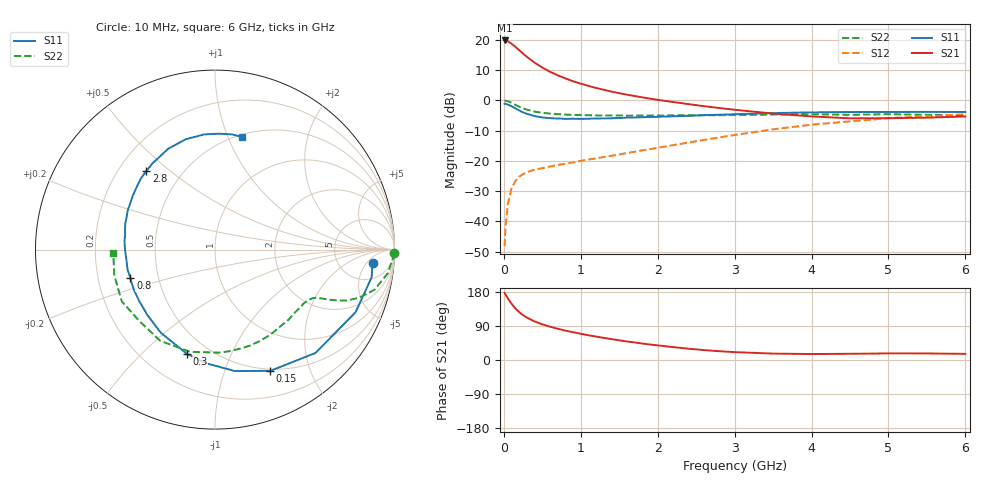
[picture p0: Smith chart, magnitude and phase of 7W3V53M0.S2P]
! Infineon Technologies  Discrete & RF Semiconductors
! BFS17W
! Si NPN RF Bipolar Junction Transistor in SOT323
! VCE = 3.5 V  IC = 3 mA
! Common Emitter S-Parameters:  August  1999
# GHz  S  MA  R  50
!  f  S11  S21  S12  S22
! GHz  MAG  ANG  MAG  ANG  MAG  ANG  MAG  ANG
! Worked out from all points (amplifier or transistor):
!   36 points, 10 MHz to 6 GHz, reference 50 ohm
!   highest |S21| = 19.9 dB at 10 MHz (marker M1)
!   |S21| within 3 dB of that: start of sweep to 190.3 MHz
!   unconditionally stable (mu >= 1): 707.7 MHz to 3.071 GHz; 4.108 GHz to end of sweep
!   at 250 MHz: K = 0.44, MSG = 19.9 dB, |S12| = -24.4 dB
!   at 1.4 GHz: K = 1.29, MAG = 7.4 dB, |S12| = -18.3 dB
!   at 6 GHz: K = 1.09, MAG = -2.2 dB, |S12| = -4.6 dB
!   S11 on the Smith chart (normalised r, x): 10 MHz: 11, -7; 150 MHz: 0.48, -1.44; 300 MHz: 0.38, -0.69; 800 MHz: 0.34, -0.14; 2.8 GHz: 0.31, +0.42; 6 GHz: 0.52, +1.13
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0.01  0.8808 -4.8  9.836 177.2  0.0039 84.2  0.9978 -1.1
0.02  0.8864 -10.0  9.808 173.3  0.0076 85.6  0.9907 -3.2
0.05  0.8574 -24.0  9.536 163.2  0.0188 76.9  0.9718 -7.8
0.1  0.8032 -45.8  8.693 148.6  0.0353 66.7  0.9166 -14.1
0.15  0.7425 -65.5  7.741 135.9  0.0468 57.9  0.8479 -18.4
0.2  0.6853 -80.8  6.788 126.2  0.0552 53.3  0.7899 -21.0
0.25  0.6358 -94.1  5.95 118.3  0.0604 48.9  0.7404 -22.5
0.3  0.6014 -105.1  5.261 111.9  0.0655 46.7  0.7052 -23.4
0.4  0.5529 -123.1  4.226 101.7  0.0716 43.9  0.6544 -24.6
0.5  0.5243 -135.9  3.508 94.1  0.076 43.9  0.6252 -25.4
0.6  0.5103 -146.0  2.983 87.8  0.0809 44.5  0.607 -26.5
0.8  0.4977 -161.4  2.319 77.6  0.0901 47.1  0.5848 -29.7
0.9  0.4997 -167.2  2.08 73.3  0.0948 48.6  0.5777 -31.4
1.1  0.4994 -177.6  1.743 65.2  0.1059 51.8  0.5705 -35.6
1.3  0.5066 174.0  1.503 58.3  0.1164 54.7  0.5647 -40.3
1.6  0.5211 163.5  1.248 48.9  0.1354 58.5  0.5619 -47.7
2.2  0.5479 146.5  0.944 34.0  0.1828 63.6  0.5674 -64.3
2.8  0.5813 131.1  0.751 23.2  0.245 64.3  0.5718 -82.2
3.5  0.6193 114.9  0.608 16.9  0.3336 60.6  0.5861 -103.7
4.5  0.6446 95.4  0.507 16.4  0.4518 48.8  0.5798 -136.6
5.5  0.6488 81.6  0.52 17.3  0.5517 36.1  0.5789 -165.6
6  0.6458 76.5  0.544 16.2  0.5906 30.0  0.5674 -178.3
